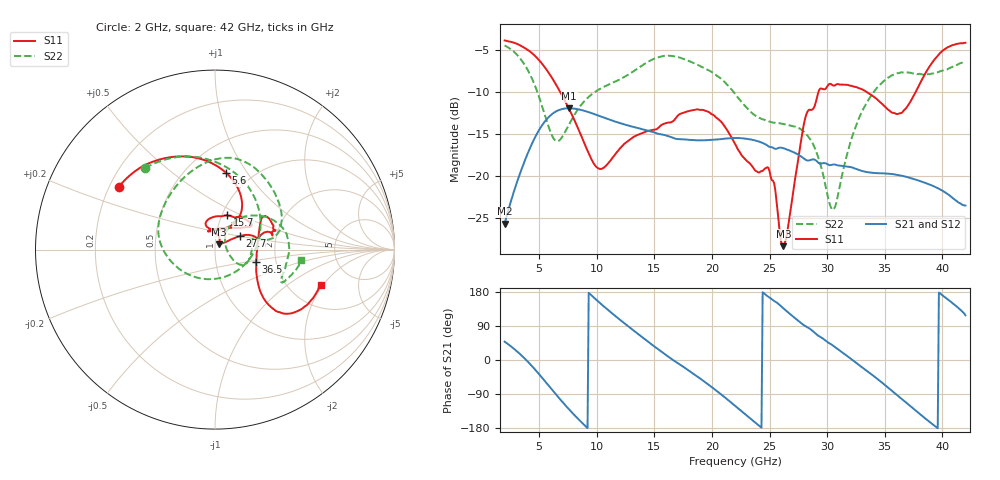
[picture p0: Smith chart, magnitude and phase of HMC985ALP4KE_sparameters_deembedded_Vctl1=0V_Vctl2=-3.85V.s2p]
!s2p File: Measurements: S11, S21, S12, S22
# GHz S dB R 50.0
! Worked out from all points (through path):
!   401 points, 2 GHz to 42 GHz, reference 50 ohm
!   highest |S21| = -11.95 dB at 7.6 GHz (marker M1); lowest = -25.7 dB at 2 GHz (marker M2)
!   lowest |S11| = -28.4 dB at 26.2 GHz (marker M3), VSWR 1.08, Z = 52.3 + j3.16 ohm
!   |S11| at or under -10 dB: 6.821 GHz to 29.25 GHz (22.43 GHz wide, 124 % of centre); 33.42 GHz to 37.69 GHz (4.271 GHz wide, 12 % of centre)
!   |S22| runs from -24.1 to -4.5 dB; largest |S21 - S12| = 0.00023
!   S11 on the Smith chart (normalised r, x): 2 GHz: 0.24, +0.28; 5.6 GHz: 0.76, +0.80; 15.7 GHz: 1.06, +0.42; 27.7 GHz: 1.30, +0.20; 36.5 GHz: 1.57, -0.23; 42 GHz: 2.95, -1.89
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2  -3.87 147.0  -25.70 48.5  -25.71 48.5  -4.46 130.6
3.6  -4.65 120.2  -18.74 8.2  -18.74 8.2  -6.49 85.2
4.6  -5.66 101.4  -15.53 -23.6  -15.53 -23.6  -9.13 48.2
5.6  -7.28 81.8  -13.34 -59.4  -13.35 -59.4  -13.22 -3.1
6.5  -9.21 66.5  -12.30 -92.3  -12.30 -92.3  -15.86 -69.3
7.6  -12.04 54.7  -11.95 -130.4  -11.95 -130.4  -13.86 -136.8
8.7  -15.39 54.9  -12.17 -165.1  -12.17 -165.1  -11.46 -171.1
10.4  -19.17 89.7  -12.95 147.1  -12.95 147.1  -9.55 161.6
15.4  -14.21 75.7  -15.01 26.9  -15.02 26.9  -5.84 86.2
15.7  -13.87 70.4  -15.08 20.2  -15.08 20.2  -5.74 82.3
19.2  -12.14 33.7  -15.76 -53.9  -15.76 -53.9  -7.08 37.0
22  -16.18 51.3  -15.49 -120.7  -15.49 -120.8  -10.23 10.6
24.9  -19.05 104.6  -16.47 166.7  -16.47 166.7  -13.49 12.9
26.2  -28.37 52.2  -16.71 136.4  -16.71 136.3  -13.84 -3.5
27.7  -16.12 28.6  -17.66 98.2  -17.65 98.2  -14.45 -24.1
28.7  -12.11 12.6  -18.05 77.7  -18.05 77.7  -16.01 -31.5
30.6  -9.26 19.6  -18.64 35.7  -18.64 35.7  -23.91 23.0
32.8  -9.58 33.9  -19.31 -14.1  -19.31 -14.2  -12.99 51.4
35.4  -12.22 11.7  -19.75 -75.6  -19.75 -75.6  -8.22 20.0
36.5  -12.47 -16.7  -19.99 -103.5  -19.99 -103.5  -7.67 6.2
39.5  -5.86 -43.7  -21.40 -177.6  -21.39 -177.6  -7.67 -25.8
42  -4.15 -18.5  -23.53 118.0  -23.53 117.9  -6.36 -6.7
